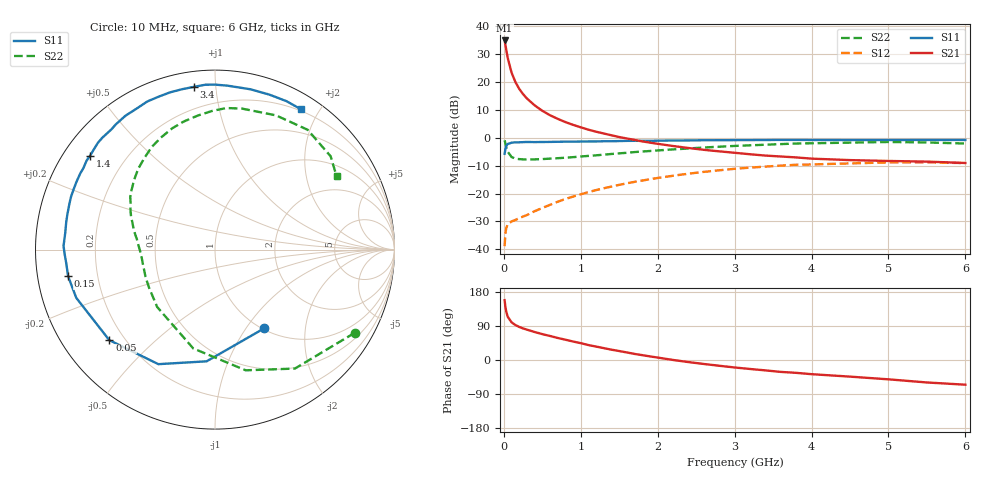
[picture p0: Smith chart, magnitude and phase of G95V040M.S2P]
! SIEMENS Small Signal Semiconductors
! BFG235
! Si NPN RF Bipolar Junction Transistor in SOT223
! VCE = 5 V  IC = 40 mA
! Common Emitter S-Parameters:  July  1994
# GHz  S  MA  R  50
!  f  S11  S21  S12  S22
! GHz  MAG  ANG  MAG  ANG  MAG  ANG  MAG  ANG
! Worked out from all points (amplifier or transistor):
!   40 points, 10 MHz to 6 GHz, reference 50 ohm
!   highest |S21| = 34.9 dB at 10 MHz (marker M1)
!   |S21| within 3 dB of that: start of sweep to 29.26 MHz
!   unconditionally stable (mu >= 1): 515 MHz to 1.278 GHz
!   at 200 MHz: K = 0.62, MSG = 23.2 dB, |S12| = -28.8 dB
!   at 1.5 GHz: K = 0.97, MSG = 8.6 dB, |S12| = -16.9 dB
!   at 6 GHz: K = 0.93, MSG = 0.0 dB, |S12| = -9.1 dB
!   S11 on the Smith chart (normalised r, x): 10 MHz: 1.02, -1.22; 50 MHz: 0.14, -0.36; 150 MHz: 0.09, -0.09; 1.4 GHz: 0.08, +0.33; 3.4 GHz: 0.08, +0.88; 6 GHz: 0.18, +1.78
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0.01  0.5174 -57.8  55.91 157.9  0.0114 68.9  0.9058 -30.8
0.02  0.6242 -94.3  47.06 140.8  0.019 54.5  0.7985 -56.1
0.03  0.712 -116.3  39.03 128.7  0.0237 45.1  0.6941 -75.7
0.05  0.7754 -139.4  27.31 114.4  0.0282 33.8  0.5639 -102.4
0.1  0.8184 -160.8  14.86 99.5  0.0316 28.2  0.454 -135.2
0.15  0.8318 -169.7  10.06 92.2  0.0337 30.3  0.4241 -150.2
0.2  0.8322 -174.7  7.557 87.3  0.0363 33.1  0.4157 -158.7
0.25  0.8383 -178.4  6.09 83.3  0.0388 36.6  0.4108 -164.2
0.3  0.8442 178.6  5.092 80.1  0.0412 39.4  0.4097 -168.5
0.4  0.8395 173.8  3.832 73.9  0.0483 44.3  0.4112 -174.2
0.5  0.8431 169.4  3.057 68.3  0.0552 47.8  0.4163 -178.3
0.6  0.8458 166.4  2.548 63.4  0.0628 49.6  0.4239 178.1
0.7  0.8504 162.5  2.196 58.2  0.0714 51.1  0.4319 174.9
0.9  0.8562 156.9  1.713 48.8  0.0884 51.2  0.4509 169.6
1.1  0.8624 150.5  1.401 39.4  0.1062 50.1  0.4746 164.1
1.4  0.8705 143.0  1.111 27.2  0.1338 46.6  0.514 156.1
2.2  0.8972 123.8  0.714 0.1  0.2091 31.4  0.6212 133.5
3.2  0.9121 101.6  0.508 -23.7  0.2923 7.5  0.7345 103.7
3.4  0.9146 97.3  0.481 -27.4  0.3052 2.4  0.7529 97.3
4.5  0.9148 77.5  0.399 -43.9  0.3481 -24.1  0.8214 65.6
5.5  0.9179 64.3  0.375 -59.3  0.3642 -46.6  0.828 38.9
6  0.917 58.4  0.354 -65.2  0.3524 -55.1  0.7909 31.1
